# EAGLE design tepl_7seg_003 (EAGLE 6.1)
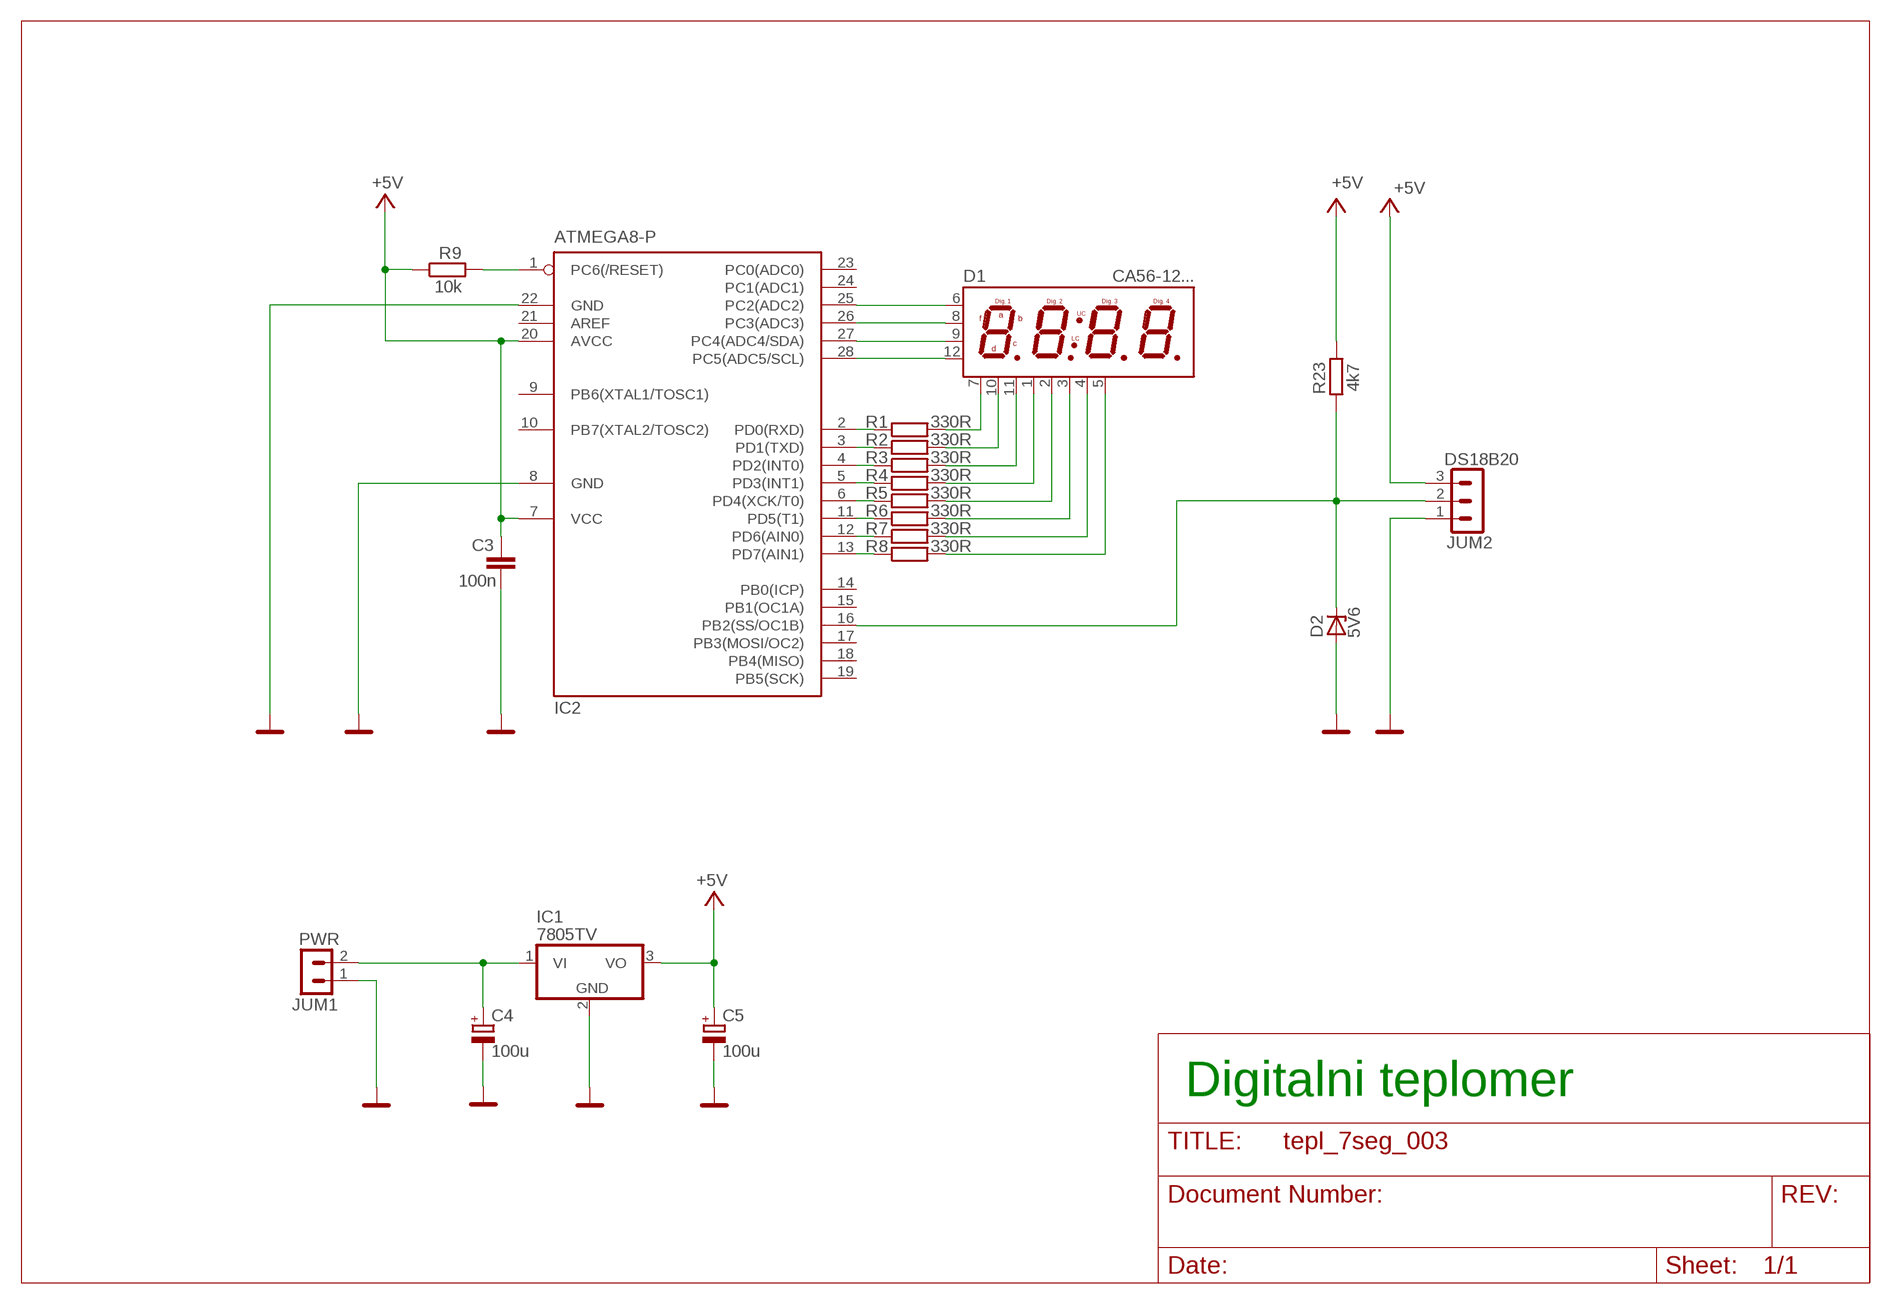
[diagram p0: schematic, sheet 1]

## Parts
C3  100n  C-EU050-024X044  [C050-024X044]
C4  100u  CPOL-EUE5-8.5  [E5-8,5]
C5  100u  CPOL-EUE5-8.5  [E5-8,5]
D1  CA56-12...  CA56-21SRWA  [CA56-21]
D2  5V6  1N821  [DO35Z10]
IC1  7805TV  [TO220V]
IC2  ATMEGA8-P  MEGA8-P  [DIL28-3]
JUM1  PWR  S1G2_JUMP  [S1G2_JUM]
JUM2  DS18B20  S1G3_JUMP  [S1G3_JUM]
R1  330R  R-EU_0207/10  [0207/10]
R2  330R  R-EU_0207/10  [0207/10]
R3  330R  R-EU_0207/10  [0207/10]
R4  330R  R-EU_0207/10  [0207/10]
R5  330R  R-EU_0207/10  [0207/10]
R6  330R  R-EU_0207/10  [0207/10]
R7  330R  R-EU_0207/10  [0207/10]
R8  330R  R-EU_0207/10  [0207/10]
R9  10k  R-EU_0207/10  [0207/10]
R23  4k7  R-EU_0207/10  [0207/10]

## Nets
+5V: C3.1 C5.+ IC1.3(VO) IC2.7(VCC) IC2.20(AVCC) JUM2.3 R9.1 R23.1
D0: D1.7 R1.2
D1: D1.10 R2.2
D2: D1.11 R3.2
D3: D1.1 R4.2
D4: D1.2 R5.2
D5: D1.3 R6.2
D6: D1.4 R7.2
D7: D1.5 R8.2
DA: D1.6 IC2.25(PC2(ADC2))
DB: D1.8 IC2.26(PC3(ADC3))
DC: D1.9 IC2.27(PC4(ADC4/SDA))
DD: D1.12 IC2.28(PC5(ADC5/SCL))
GND: C3.2 C4.- C5.- D2.A IC1.2(GND) IC2.8(GND) IC2.22(GND) JUM1.1 JUM2.1
N$1: IC2.4(PD2(INT0)) R3.1
N$2: IC2.5(PD3(INT1)) R4.1
N$3: IC2.6(PD4(XCK/T0)) R5.1
N$4: IC2.11(PD5(T1)) R6.1
N$5: IC2.12(PD6(AIN0)) R7.1
N$6: IC2.13(PD7(AIN1)) R8.1
N$7: IC2.3(PD1(TXD)) R2.1
N$8: IC2.2(PD0(RXD)) R1.1
N$9: D2.C IC2.16(PB2(SS/OC1B)) JUM2.2 R23.2
N$21: IC2.1(PC6(/RESET)) R9.2
N$28: C4.+ IC1.1(VI) JUM1.2
Unconnected: IC2.9(PB6(XTAL1/TOSC1)) IC2.10(PB7(XTAL2/TOSC2)) IC2.14(PB0(ICP)) IC2.15(PB1(OC1A)) IC2.17(PB3(MOSI/OC2)) IC2.18(PB4(MISO)) IC2.19(PB5(SCK)) IC2.21(AREF) IC2.23(PC0(ADC0)) IC2.24(PC1(ADC1))

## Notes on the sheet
- Digitalni teplomer

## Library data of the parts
C3 = rcl:C-EU: CAPACITOR, European symbol
C4 C5 = rcl:CPOL-EU: POLARIZED CAPACITOR, European symbol
D1 = &my:CA56-21SRWA; IO: CA56-21SRWA
D2 = diode:1N821: Reference DIODE
IC1 = linear:78*: Positive VOLTAGE REGULATOR Source: http://cache.national.com/ds/LM/LM78L05.pdf http://www.fairchildsemi.com/ds/LM/LM7805.pdf
IC2 = atmel:MEGA8-P: MICROCONTROLLER 8 Kbytes FLASH, 1 kbytes SRAM, 512 bytes EEPROM, USART, 4-channel 10 bit ADC, 2-channel 8 bit ADC Pin compatible with Atmega48, ATMega88, ATMega168 Source: avr.lbr
JUM1 = #PaJa_konektory:S1G2_JUMP: Radove konektory - koliky - 2x
JUM2 = #PaJa_konektory:S1G3_JUMP: Radove konektory - koliky - 3x
R1-R9 R23 = rcl:R-EU_: RESISTOR, European symbol

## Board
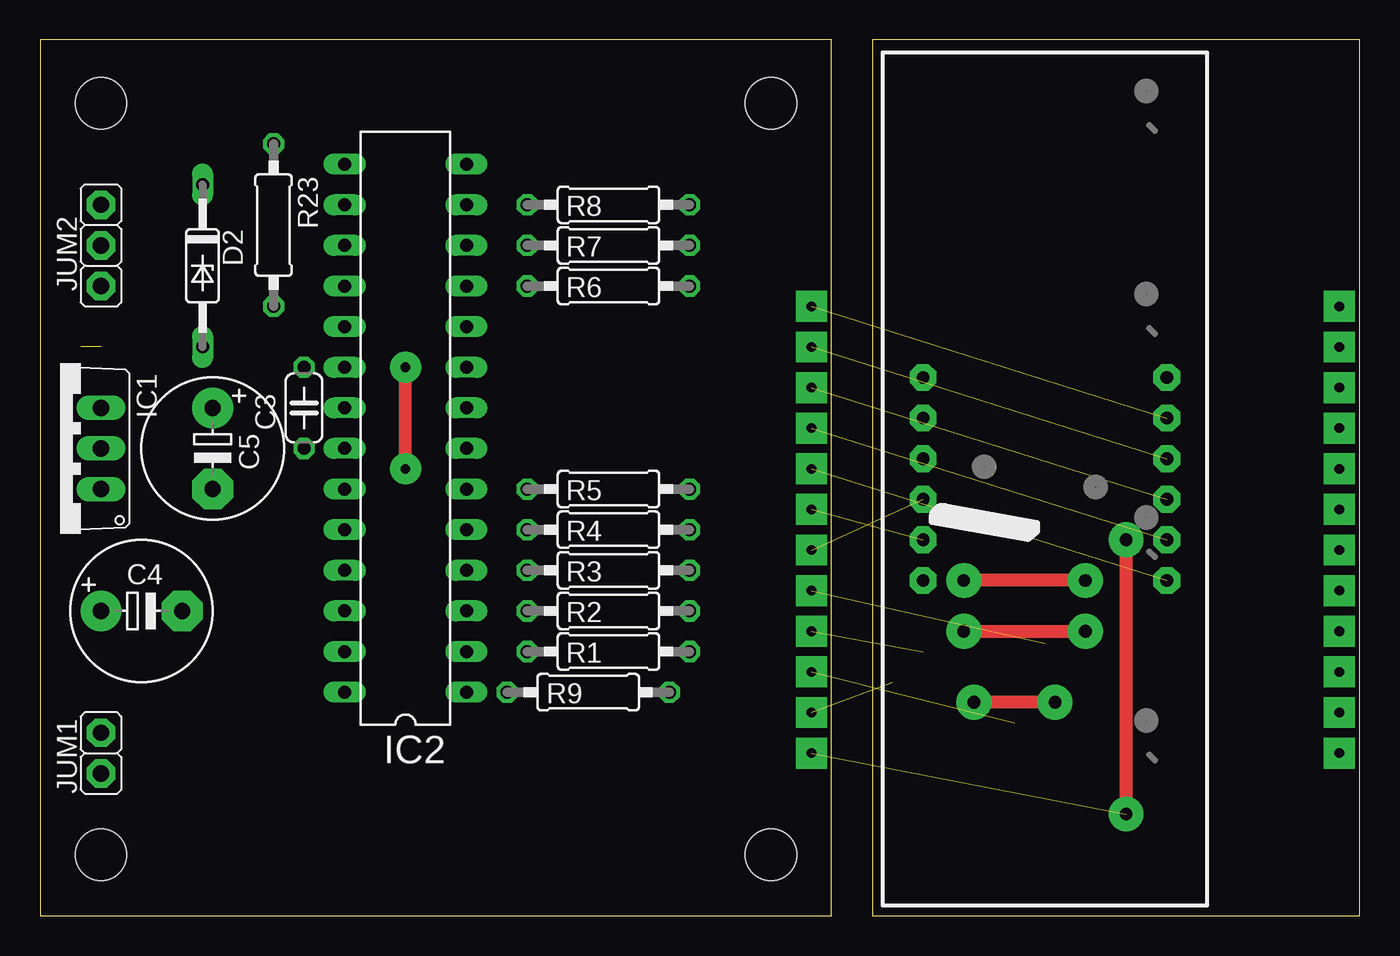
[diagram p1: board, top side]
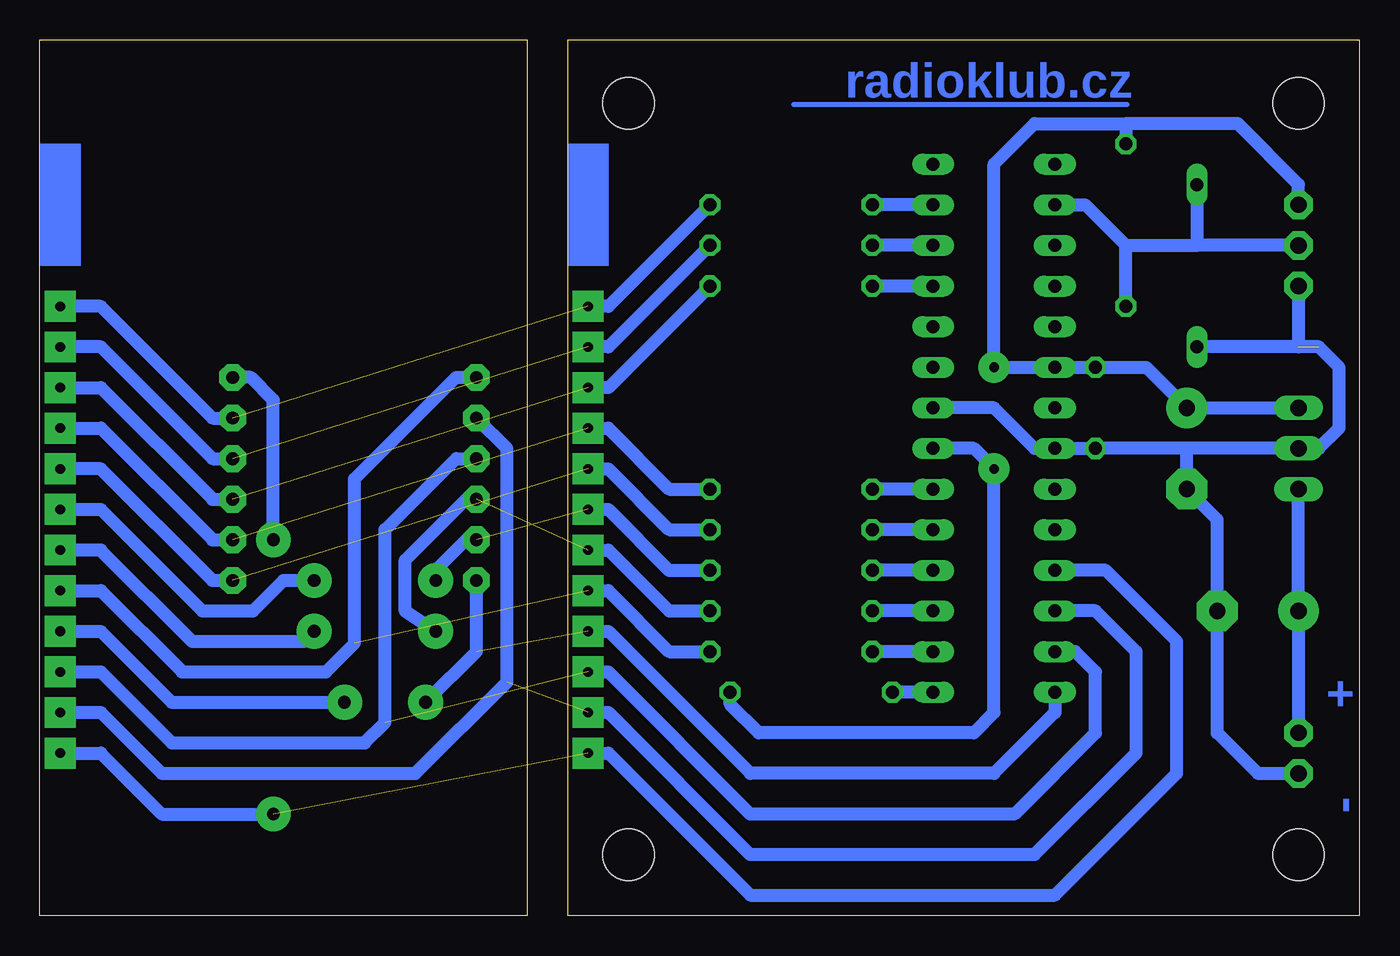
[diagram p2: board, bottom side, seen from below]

Size 82.55 x 54.76 mm. Coordinates in mm from the lower left corner, seen from the top.
Outline: 0,0 49.51,0 49.51,54.76 0,54.76 0,0
Outline: 82.55,54.76 52.07,54.76 52.07,0 82.55,0 82.55,54.76
Copper layers (1*16): Top 0.035mm / dielectric 1.5mm / Bottom 0.035mm
Design rules: minimum track width 10mil, minimum drill 24mil, track to track 8mil, track to pad 8mil, pad to pad 8mil, via to via 8mil, smd to smd 8mil, copper to edge 40mil, drill to drill 8mil, minimum pad ring 10mil, minimum via ring 8mil, stop-mask expansion 4mil, vias tented up to drill 0mil, thermal gap 10mil
Holes 3.2 mm at 3.81,50.8 45.72,50.8 45.72,3.81 3.81,3.81

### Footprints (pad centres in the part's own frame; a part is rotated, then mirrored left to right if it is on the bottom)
C050-024X044 = drill 0.813 octagon: 1 -2.54,0; 2 2.54,0
E5-8,5 = drill 1.016 pad 2.54: + -2.54,0 | drill 1.016 pad 2.54 octagon: - 2.54,0
CA56-21 = drill 0.8 pad 1.676 octagon: 1 -6.35,-7.62; 2 -3.81,-7.62; 3 -1.27,-7.62; 4 1.27,-7.62; 5 3.81,-7.62; 6 6.35,-7.62; 7 6.35,7.62; 8 3.81,7.62; 9 1.27,7.62; 10 -1.27,7.62; 11 -3.81,7.62; 12 -6.35,7.62
DO35Z10 = drill 0.813 long: A 5.08,0; C -5.08,0
TO220V = drill 1.016 long: 1 -2.54,-2.54; 2 0,-2.54; 3 2.54,-2.54
DIL28-3 = drill 0.813 long: 1 -16.51,-3.81; 2 -13.97,-3.81; 3 -11.43,-3.81; 4 -8.89,-3.81; 5 -6.35,-3.81; 6 -3.81,-3.81; 7 -1.27,-3.81; 8 1.27,-3.81; 9 3.81,-3.81; 10 6.35,-3.81; 11 8.89,-3.81; 12 11.43,-3.81; 13 13.97,-3.81; 14 16.51,-3.81; 15 16.51,3.81; 16 13.97,3.81; 17 11.43,3.81; 18 8.89,3.81; 19 6.35,3.81; 20 3.81,3.81; 21 1.27,3.81; 22 -1.27,3.81; 23 -3.81,3.81; 24 -6.35,3.81; 25 -8.89,3.81; 26 -11.43,3.81; 27 -13.97,3.81; 28 -16.51,3.81
S1G2_JUM = drill 1.016 pad 1.778 octagon: 1 -1.27,0; 2 1.27,0
S1G3_JUM = drill 1.016 pad 1.778 octagon: 1 -2.54,0; 2 0,0; 3 2.54,0
0207/10 = drill 0.813 octagon: 1 -5.08,0; 2 5.08,0

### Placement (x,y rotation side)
C3  16.51,31.75 270 top
C4  6.35,19.05 0 top
C5  10.79,29.21 270 top
D1  62.87,27.3 90 top
D2  10.16,40.64 270 top
IC1  1.27,29.21 90 top
IC2  22.86,30.48 90 top
JUM1  3.81,10.16 90 top
JUM2  3.81,41.91 90 top
R1  35.56,16.51 0 top
R2  35.56,19.05 0 top
R3  35.56,21.59 0 top
R4  35.56,24.13 0 top
R5  35.56,26.67 0 top
R6  35.56,39.37 0 top
R7  35.56,41.91 0 top
R8  35.56,44.45 0 top
R9  34.29,13.97 180 top
R23  14.61,43.18 270 top

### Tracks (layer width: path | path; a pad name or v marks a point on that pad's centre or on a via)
+5V  (via drill 0.6 pad 1.93)
  Top 0.813: v22.86,27.94 v22.86,34.29
  Bottom 0.813: v22.86,27.94 22.86,12.7 24.13,11.43 37.57,11.43 39.37,13.23 R9.1 | v22.86,27.94 22.86,27.41 | IC2.7 24.13,29.21 v22.86,27.94 | IC1.3 C5.+ 13.34,34.29 C3.1 IC2.20 v22.86,34.29 22.86,46.99 20.32,49.53 14.61,49.53 | 14.61,49.53 R23.1 | 14.61,49.53 7.62,49.53 3.81,45.72 JUM2.3
D0  (via drill 0.6 pad 1.93)  (1 unrouted)
  Bottom 0.813: D1.7 56.52,33.66 62.87,27.3 62.87,17.04 64.66,15.24 73.66,15.24 78.74,20.32 v81.28,20.32 | 48.26,20.32 46.99,20.32 43.18,16.51 R1.2
D1  (via drill 0.6 pad 1.93, 0.8 pad 2.18)  (1 unrouted)
  Top 0.813: v57.78,17.78 v65.41,17.78
  Bottom 0.813: D1.10 55.88,26.04 59.69,22.23 59.69,19.05 v57.78,17.78 | v65.41,17.78 66.04,17.14 73.03,17.14 78.74,22.86 v81.28,22.86 | 48.26,22.86 46.99,22.86 43.18,19.05 R2.2
D2  (via drill 0.6 pad 1.93, 0.8 pad 2.18)  (1 unrouted)
  Top 0.813: v65.41,20.95 v57.78,20.95
  Bottom 0.813: D1.11 55.88,23.5 57.78,21.59 v57.78,20.95 | v65.41,20.95 67.31,20.95 69.22,19.05 72.39,19.05 78.74,25.4 v81.28,25.4 | 48.26,25.4 46.99,25.4 43.18,21.59 R3.2
D3  (via drill 0.6 pad 1.93)  (1 unrouted)
  Bottom 0.813: D1.1 71.75,20.95 78.74,27.94 v81.28,27.94 | 48.26,27.94 46.99,27.94 43.18,24.13 R4.2
D4  (via drill 0.6 pad 1.93)  (1 unrouted)
  Bottom 0.813: v81.28,30.48 78.74,30.48 71.75,23.5 D1.2 | 48.26,30.48 46.99,30.48 43.18,26.67 R5.2
D5  (via drill 0.6 pad 1.93)  (1 unrouted)
  Bottom 0.813: R6.2 46.99,33.02 48.26,33.02 | v81.28,33.02 78.74,33.02 71.75,26.04 D1.3
D6  (via drill 0.6 pad 1.93)  (1 unrouted)
  Bottom 0.813: R7.2 46.99,35.56 48.26,35.56 | v81.28,35.56 78.74,35.56 71.75,28.57 D1.4
D7  (via drill 0.6 pad 1.93)  (1 unrouted)
  Bottom 0.813: R8.2 46.99,38.1 48.26,38.1 | v81.28,38.1 78.74,38.1 71.75,31.11 D1.5
DA  (via drill 0.6 pad 1.93, 0.8 pad 2.18)  (1 unrouted)
  Top 0.813: v67.94,6.35 v67.94,23.5
  Bottom 0.813: IC2.25 15.88,21.59 11.43,17.14 11.43,8.89 19.05,1.27 38.1,1.27 46.99,10.16 48.26,10.16 | v67.94,23.5 67.94,32.23 69.36,33.66 D1.6 | v81.28,10.16 78.74,10.16 74.93,6.35 v67.94,6.35
DB  (via drill 0.6 pad 1.93)  (1 unrouted)
  Bottom 0.813: IC2.26 16.51,19.05 13.97,16.51 13.97,10.16 20.32,3.81 38.1,3.81 46.99,12.7 48.26,12.7 | D1.8 53.34,29.21 53.34,14.61 59.05,8.89 74.93,8.89 78.74,12.7 v81.28,12.7
DC  (via drill 0.6 pad 1.93)  (1 unrouted)
  Bottom 0.813: IC2.27 17.78,16.51 16.51,15.24 16.51,11.43 21.59,6.35 38.1,6.35 46.99,15.24 48.26,15.24 | D1.9 56.52,28.57 60.96,24.13 60.96,12.06 62.23,10.79 74.3,10.79 78.74,15.24 v81.28,15.24
DD  (via drill 0.6 pad 1.93, 0.8 pad 2.18)  (1 unrouted)
  Top 0.813: v63.5,13.34 v58.42,13.34
  Bottom 0.813: IC2.28 19.05,12.7 22.86,8.89 38.1,8.89 46.99,17.78 48.26,17.78 | D1.12 55.24,16.51 v58.42,13.34 | v81.28,17.78 78.74,17.78 74.3,13.34 v63.5,13.34
GND  (1 unrouted)
  Bottom 0.813: IC2.8 22.86,31.75 20.32,29.21 IC2.22 C3.2 10.79,29.21 | 10.79,29.21 IC1.2 2.54,29.21 1.27,30.48 1.27,34.29 2.54,35.56 3.81,35.56 | 10.79,29.21 C5.- 8.89,24.77 C4.- 8.89,11.43 6.35,8.89 JUM1.1 | 3.81,35.56 D2.A | JUM2.1 3.81,35.56
N$1
  Bottom 0.813: IC2.4 R3.1
N$2
  Bottom 0.813: IC2.5 R4.1
N$3
  Bottom 0.813: IC2.6 R5.1
N$4
  Bottom 0.813: IC2.11 R6.1
N$5
  Bottom 0.813: IC2.12 R7.1
N$6
  Bottom 0.813: IC2.13 R8.1
N$7
  Bottom 0.813: IC2.3 R2.1
N$8
  Bottom 0.813: IC2.2 R1.1
N$9
  Bottom 0.813: IC2.16 17.14,44.45 14.61,41.91 | 14.61,41.91 10.16,41.91 | R23.2 14.61,41.91 | D2.C 10.16,41.91 | JUM2.2 10.16,41.91
N$21
  Bottom 0.813: IC2.1 R9.2
N$28
  Bottom 0.813: IC1.1 C4.+ JUM1.2
N$29  (via drill 0.6 pad 1.93)
  other vias: 48.26,38.1
N$30  (via drill 0.6 pad 1.93)
  other vias: 48.26,35.56
N$31  (via drill 0.6 pad 1.93)
  other vias: 48.26,33.02
N$33  (via drill 0.6 pad 1.93)
  other vias: 48.26,30.48
N$34  (via drill 0.6 pad 1.93)
  other vias: 48.26,27.94
N$35  (via drill 0.6 pad 1.93)
  other vias: 48.26,25.4
N$36  (via drill 0.6 pad 1.93)
  other vias: 48.26,22.86
N$37  (via drill 0.6 pad 1.93)
  other vias: 48.26,20.32
N$38  (via drill 0.6 pad 1.93)
  other vias: 48.26,17.78
N$39  (via drill 0.6 pad 1.93)
  other vias: 48.26,15.24
N$40  (via drill 0.6 pad 1.93)
  other vias: 48.26,12.7
N$41  (via drill 0.6 pad 1.93)
  other vias: 48.26,10.16
S$1
  Bottom 0.305: 14.53,50.71 35.39,50.71
(copper drawn outside any net)
  shapes: Bottom area x2

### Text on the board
Bottom: radioklub.cz | + | -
